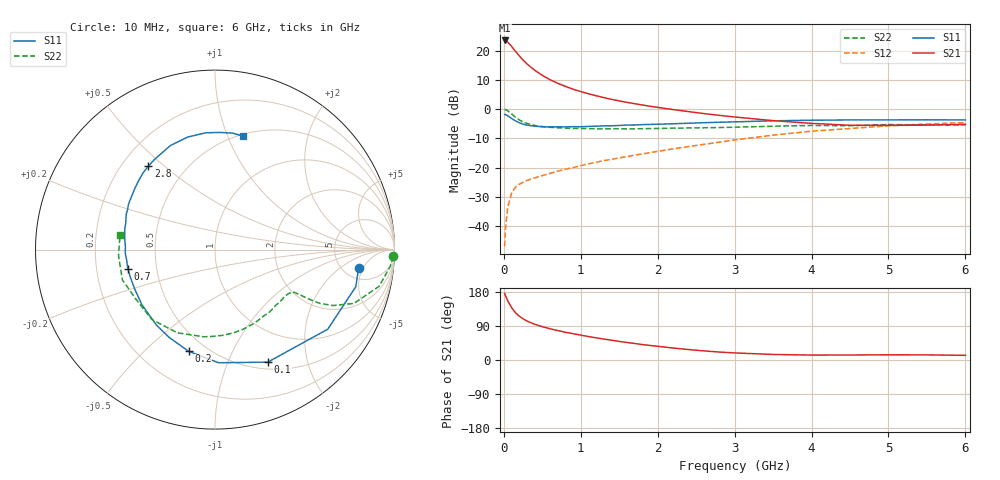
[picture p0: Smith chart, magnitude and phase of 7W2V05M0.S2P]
! Infineon Technologies  Discrete & RF Semiconductors
! BFS17W
! Si NPN RF Bipolar Junction Transistor in SOT323
! VCE = 2 V  IC = 5 mA
! Common Emitter S-Parameters:  August  1999
# GHz  S  MA  R  50
!  f  S11  S21  S12  S22
! GHz  MAG  ANG  MAG  ANG  MAG  ANG  MAG  ANG
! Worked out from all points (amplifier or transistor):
!   36 points, 10 MHz to 6 GHz, reference 50 ohm
!   highest |S21| = 23.5 dB at 10 MHz (marker M1)
!   |S21| within 3 dB of that: start of sweep to 129.8 MHz
!   unconditionally stable (mu >= 1): 531.1 MHz to 3.406 GHz; 3.652 GHz to end of sweep
!   at 250 MHz: K = 0.60, MSG = 20.9 dB, |S12| = -25.1 dB
!   at 1.4 GHz: K = 1.28, MAG = 7.1 dB, |S12| = -17.2 dB
!   at 6 GHz: K = 1.10, MAG = -2.2 dB, |S12| = -4.6 dB
!   S11 on the Smith chart (normalised r, x): 10 MHz: 6.93, -4.07; 100 MHz: 0.58, -1.41; 200 MHz: 0.40, -0.69; 700 MHz: 0.34, -0.10; 2.8 GHz: 0.31, +0.44; 6 GHz: 0.52, +1.13
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0.01  0.8068 -7.3  14.98 175.7  0.0045 82.3  0.9923 -2.2
0.02  0.8111 -14.8  14.96 170.4  0.0087 85.5  0.9815 -5.4
0.05  0.769 -35.2  14.03 156.7  0.0207 73.0  0.9371 -12.6
0.1  0.6926 -64.9  11.88 138.5  0.0362 60.0  0.8299 -21.2
0.15  0.6307 -88.2  9.816 125.0  0.046 52.8  0.7268 -25.4
0.2  0.5853 -104.6  8.18 115.7  0.0518 49.3  0.6547 -27.2
0.25  0.5519 -117.5  6.905 108.6  0.0556 46.9  0.6031 -27.7
0.3  0.5324 -127.8  5.954 103.0  0.06 46.3  0.5696 -27.9
0.4  0.5101 -143.0  4.638 94.3  0.0663 47.0  0.525 -28.1
0.5  0.4985 -153.5  3.788 87.9  0.0726 48.7  0.5025 -28.3
0.6  0.4961 -161.5  3.189 82.4  0.0794 50.4  0.4882 -29.2
0.7  0.4973 -167.7  2.771 77.7  0.0866 52.3  0.4787 -30.7
0.9  0.5003 -177.6  2.194 69.4  0.0998 55.0  0.4657 -34.5
1.1  0.5054 173.9  1.831 61.8  0.1157 57.1  0.4631 -39.2
1.3  0.5165 166.7  1.574 55.2  0.1313 58.6  0.4584 -44.5
1.6  0.5329 158.1  1.304 46.2  0.1539 60.2  0.4589 -52.8
2.2  0.5612 142.9  0.982 31.6  0.2086 61.9  0.4717 -71.4
2.8  0.5952 128.6  0.782 21.0  0.2717 60.5  0.4837 -91.2
3.5  0.6307 113.2  0.635 14.6  0.3583 55.7  0.509 -114.4
4.5  0.6529 94.6  0.529 13.2  0.4658 43.8  0.5202 -148.2
5.5  0.6562 81.5  0.531 13.5  0.5545 31.8  0.5388 -176.3
6  0.6519 76.3  0.55 12.3  0.5899 26.0  0.5355 171.4
